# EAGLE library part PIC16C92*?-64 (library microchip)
MICROCONTROLLER with LCD driver
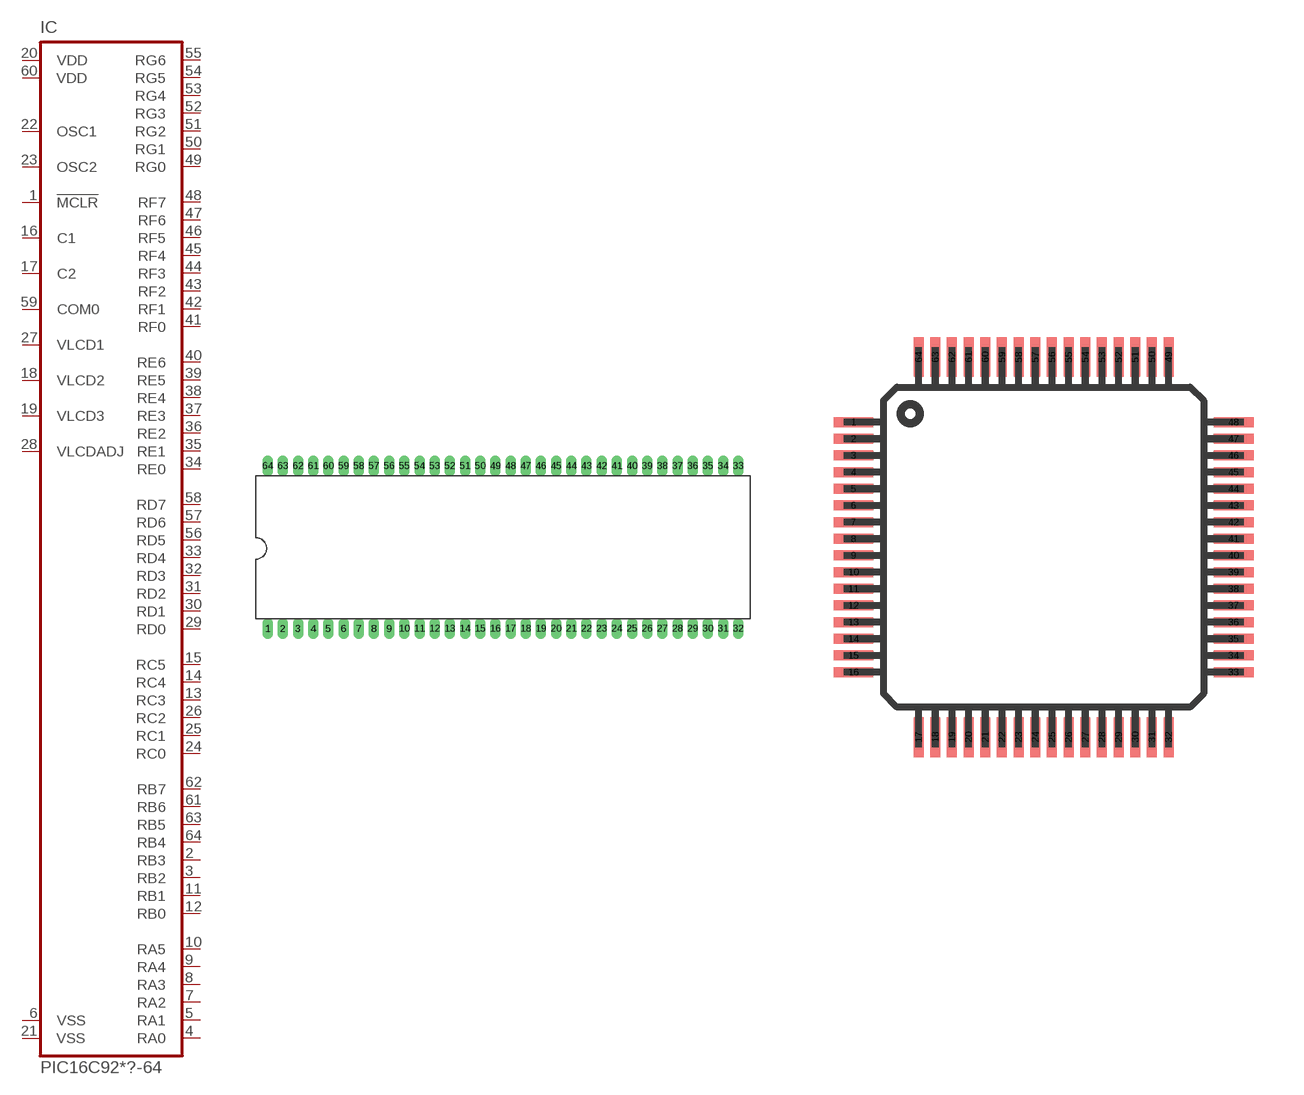
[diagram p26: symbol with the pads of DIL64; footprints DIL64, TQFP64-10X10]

Designator prefix IC

## PIC16C923PS-64 (OC_FARNELL: unknown; OC_NEWARK: unknown), PIC16C924PS-64 (OC_FARNELL: unknown; OC_NEWARK: unknown)  [DIL64]
1  !MCLR  in
2  RB3
3  RB2
4  RA0
5  RA1
6  VSS  pwr
7  RA2
8  RA3
9  RA4
10  RA5
11  RB1
12  RB0
13  RC3
14  RC4
15  RC5
16  C1  in
17  C2  in
18  VLCD2  in
19  VLCD3  in
20  VDD  pwr
21  VSS  pwr
22  OSC1  in
23  OSC2  out
24  RC0
25  RC1
26  RC2
27  VLCD1  in
28  VLCDADJ  in
29  RD0
30  RD1
31  RD2
32  RD3
33  RD4
34  RE0
35  RE1
36  RE2
37  RE3
38  RE4
39  RE5
40  RE6
41  RF0
42  RF1
43  RF2
44  RF3
45  RF4
46  RF5
47  RF6
48  RF7
49  RG0
50  RG1
51  RG2
52  RG3
53  RG4
54  RG5
55  RG6
56  RD5
57  RD6
58  RD7
59  COM0  out
60  VDD  pwr
61  RB6
62  RB7
63  RB5
64  RB4

## PIC16C923TQ-64 (MF: MICROCHIP; MPN: PIC16C923-04I/PT; OC_FARNELL: unknown; OC_NEWARK: 23C4930), PIC16C924TQ-64 (OC_FARNELL: unknown; OC_NEWARK: unknown)  [TQFP64-10X10]
1  RA4
2  RA5
3  RB1
4  RB0
5  RC3
6  RC4
7  RC5
8  C1  in
9  C2  in
10  VLCD2  in
11  VLCD3  in
12  VDD  pwr
13  VSS  pwr
14  OSC1  in
15  OSC2  out
16  RC0
17  RC1
18  RC2
19  VLCD1  in
20  VLCDADJ  in
21  RD0
22  RD1
23  RD2
24  RD3
25  RD4
26  RE0
27  RE1
28  RE2
29  RE3
30  RE4
31  RE5
32  RE6
33  RF0
34  RF1
35  RF2
36  RF3
37  RF4
38  RF5
39  RF6
40  RF7
41  RG0
42  RG1
43  RG2
44  RG3
45  RG4
46  RG5
47  RG6
48  RD5
49  RD6
50  RD7
51  COM0  out
52  VDD  pwr
53  RB6
54  RB7
55  RB5
56  RB4
57  !MCLR  in
58  RB3
59  RB2
60  RA0
61  RA1
62  VSS  pwr
63  RA2
64  RA3

## Footprint DIL64 (pad centres in mm)
Dual In Line package type P
drill 0.711 long: 1 -27.559,-9.525; 2 -25.781,-9.525; 3 -24.003,-9.525; 4 -22.225,-9.525; 5 -20.447,-9.525; 6 -18.669,-9.525; 7 -16.891,-9.525; 8 -15.113,-9.525; 9 -13.335,-9.525; 10 -11.557,-9.525; 11 -9.779,-9.525; 12 -8.001,-9.525; 13 -6.223,-9.525; 14 -4.445,-9.525; 15 -2.667,-9.525; 16 -0.889,-9.525; 17 0.889,-9.525; 18 2.667,-9.525; 19 4.445,-9.525; 20 6.223,-9.525; 21 8.001,-9.525; 22 9.779,-9.525; 23 11.557,-9.525; 24 13.335,-9.525; 25 15.113,-9.525; 26 16.891,-9.525; 27 18.669,-9.525; 28 20.447,-9.525; 29 22.225,-9.525; 30 24.003,-9.525; 31 25.781,-9.525; 32 27.559,-9.525; 33 27.559,9.525; 34 25.781,9.525; 35 24.003,9.525; 36 22.225,9.525; 37 20.447,9.525; 38 18.669,9.525; 39 16.891,9.525; 40 15.113,9.525; 41 13.335,9.525; 42 11.557,9.525; 43 9.779,9.525; 44 8.001,9.525; 45 6.223,9.525; 46 4.445,9.525; 47 2.667,9.525; 48 0.889,9.525; 49 -0.889,9.525; 50 -2.667,9.525; 51 -4.445,9.525; 52 -6.223,9.525; 53 -8.001,9.525; 54 -9.779,9.525; 55 -11.557,9.525; 56 -13.335,9.525; 57 -15.113,9.525; 58 -16.891,9.525; 59 -18.669,9.525; 60 -20.447,9.525; 61 -22.225,9.525; 62 -24.003,9.525; 63 -25.781,9.525; 64 -27.559,9.525

## Footprint TQFP64-10X10 (pad centres in mm)
Thin Quad Flat Pack package type TQ
smd 1.2 x 0.3: 1 -5.7,3.75; 2 -5.7,3.25; 3 -5.7,2.75; 4 -5.7,2.25; 5 -5.7,1.75; 6 -5.7,1.25; 7 -5.7,0.75; 8 -5.7,0.25; 9 -5.7,-0.25; 10 -5.7,-0.75; 11 -5.7,-1.25; 12 -5.7,-1.75; 13 -5.7,-2.25; 14 -5.7,-2.75; 15 -5.7,-3.25; 16 -5.7,-3.75; 33 5.7,-3.75; 34 5.7,-3.25; 35 5.7,-2.75; 36 5.7,-2.25; 37 5.7,-1.75; 38 5.7,-1.25; 39 5.7,-0.75; 40 5.7,-0.25; 41 5.7,0.25; 42 5.7,0.75; 43 5.7,1.25; 44 5.7,1.75; 45 5.7,2.25; 46 5.7,2.75; 47 5.7,3.25; 48 5.7,3.75
smd 0.3 x 1.2: 17 -3.75,-5.7; 18 -3.25,-5.7; 19 -2.75,-5.7; 20 -2.25,-5.7; 21 -1.75,-5.7; 22 -1.25,-5.7; 23 -0.75,-5.7; 24 -0.25,-5.7; 25 0.25,-5.7; 26 0.75,-5.7; 27 1.25,-5.7; 28 1.75,-5.7; 29 2.25,-5.7; 30 2.75,-5.7; 31 3.25,-5.7; 32 3.75,-5.7; 49 3.75,5.7; 50 3.25,5.7; 51 2.75,5.7; 52 2.25,5.7; 53 1.75,5.7; 54 1.25,5.7; 55 0.75,5.7; 56 0.25,5.7; 57 -0.25,5.7; 58 -0.75,5.7; 59 -1.25,5.7; 60 -1.75,5.7; 61 -2.25,5.7; 62 -2.75,5.7; 63 -3.25,5.7; 64 -3.75,5.7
